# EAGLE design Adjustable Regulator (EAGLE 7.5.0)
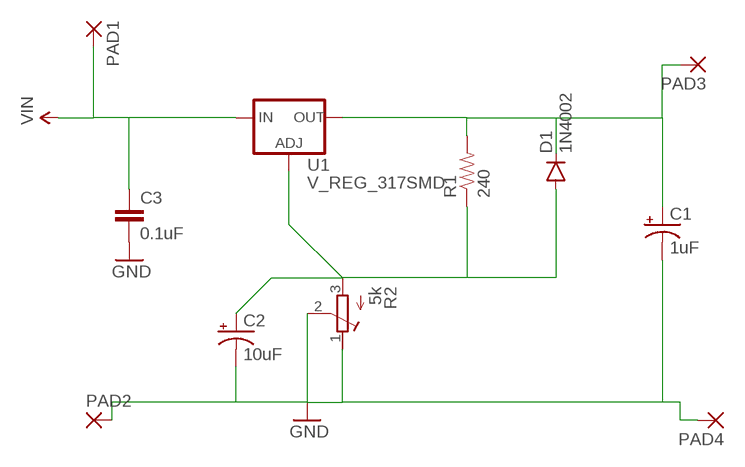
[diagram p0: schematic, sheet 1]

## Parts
C1  1uF  CAP_POLC  [PANASONIC_C]
C2  10uF  CAP_POLC  [PANASONIC_C]
C3  0.1uF  0.1UF-25V(+80/-20%)(0603)  [0603-CAP]
D1  1N4002  DIODESMB  [SMB-DIODE]
PAD1  SMD2  [SMD1,27-2,54]
PAD2  SMD2  [SMD1,27-2,54]
PAD3  SMD2  [SMD1,27-2,54]
PAD4  SMD2  [SMD1,27-2,54]
R1  240  RESISTOR0805-RES  [0805]
R2  5k  R-TRIMMT93YB  [RTRIMT93YB]
U1  V_REG_317SMD  [SOT223]

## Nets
GND: C1.- C2.- C3.2 PAD2.1(P) PAD4.1(P) R2.1(E) R2.2(S)
N$1: C2.+ D1.A R1.1 R2.3(A) U1.1(ADJ)
N$3: C1.+ D1.C PAD3.1(P) R1.2 U1.2(OUT)
VIN: C3.1 PAD1.1(P) U1.3(IN)

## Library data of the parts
C1 C2 = SparkFun-Capacitors:CAP_POL: Capacitor Polarized
C3 = SparkFun-Capacitors:0.1UF-25V(+80/-20%)(0603): CAP-00810; PROD_ID: CAP-00810
D1 = SparkFun-DiscreteSemi:DIODE: Diode; PROD_ID: DIO-09646
PAD1-PAD4 = wirepad:SMD2: SMD PAD
R1 = SparkFun-Passives:RESISTOR: Resistor
R2 = resistor:R-TRIMM: Trimm resistor
U1 = SparkFun-PowerIC:V_REG_317: Voltage Regulator Standard LM317 adjustable voltage regulator. AOI (Adjust Output Input). Google 'LM317 Calculator' for easy to use app to get the two resistor values needed. 240/720 for 5V output. 240/390 for 3.3V output. Spark Fun Electronics SKU : COM-00527

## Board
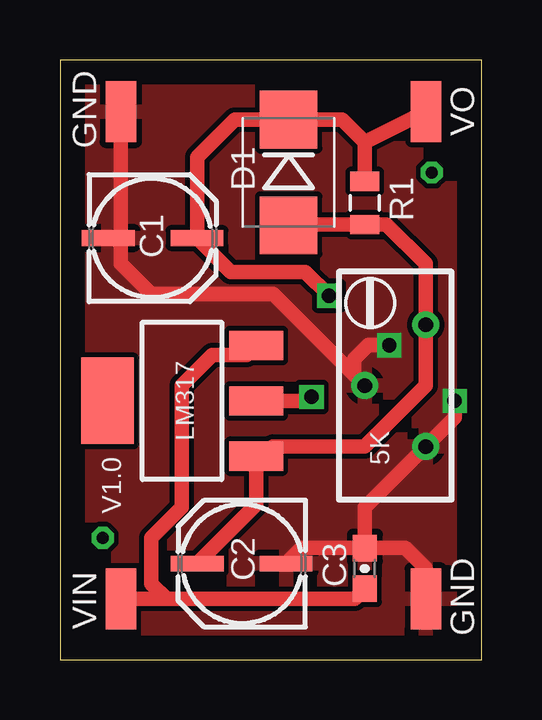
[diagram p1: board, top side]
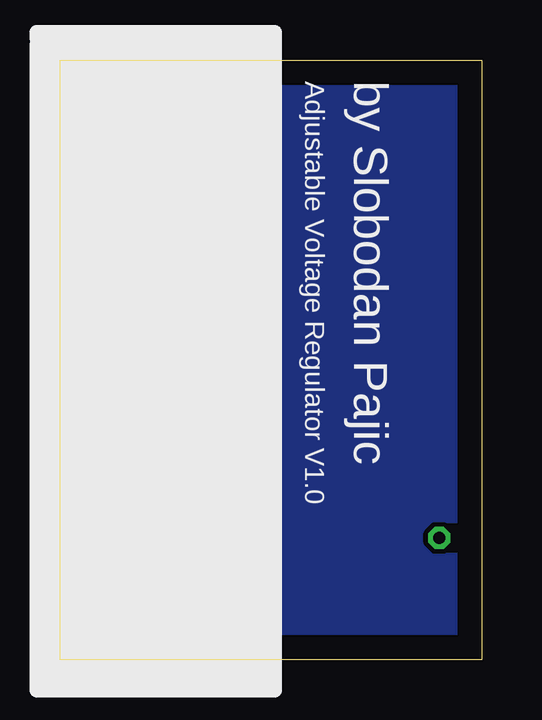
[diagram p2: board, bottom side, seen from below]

Size 17.58 x 25.01 mm. Coordinates in mm from the lower left corner, seen from the top.
Outline: 0,0 17.58,0 17.58,25.01 0,25.01 0,0
Copper layers (1*16): Top 0.035mm / dielectric 1.5mm / Bottom 0.035mm
Design rules "default": minimum track width 10mil, minimum drill 24mil, track to track 8mil, track to pad 8mil, pad to pad 8mil, via to via 8mil, smd to smd 8mil, copper to edge 40mil, drill to drill 8mil, minimum pad ring 10mil, minimum via ring 8mil, stop-mask expansion 4mil, vias tented up to drill 0mil, thermal gap 10mil

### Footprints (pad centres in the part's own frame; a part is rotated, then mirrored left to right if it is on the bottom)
PANASONIC_C = smd 2.2 x 0.65: + 1.9,-0.2; - -1.8,-0.2
0603-CAP = smd 1.1 x 1: 1 -0.85,0; 2 0.85,0
SMB-DIODE = smd 2.4 x 2.4: A 2.2,0; C -2.2,0
SMD1,27-2,54 = smd 1.27 x 2.54: 1 0,0
0805 = smd 0.8 x 1.2: 1 -0.9,0; 2 0.9,0
RTRIMT93YB = drill 0.61: 1 1.27,-2.54; 2 -1.27,0; 3 1.27,2.54
SOT223 = smd 1.219 x 2.235: 1 -2.311,-3.099; 2 0,-3.099; 3 2.311,-3.099 | smd 3.6 x 2.2: 4 0,3.099

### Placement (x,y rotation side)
C1  3.81,17.78 0 top
C2  7.62,3.81 180 top
C3  12.7,3.81 90 top
D1  9.53,20.32 270 top
PAD1  2.54,2.54 0 top
PAD2  15.24,2.54 0 top
PAD3  15.24,22.86 0 top
PAD4  2.54,22.86 0 top
R1  12.7,19.05 90 top
R2  13.97,11.43 0 top
U1  5.08,10.79 90 top

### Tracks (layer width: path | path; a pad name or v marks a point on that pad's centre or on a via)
GND  (via drill 0.6)
  Top 0.61: C3.2 14.39,4.66 15.24,3.81 PAD2.1 | C2.- 10.07,4.66 C3.2 | C3.2 12.7,6.35 R2.1 16.44,10.09 v16.44,10.79 | PAD4.1 2.54,17.78 | 2.54,17.78 2.34,17.58 C1.- | 2.54,17.78 2.54,16.51 3.81,15.24 8.89,15.24 12.27,11.87 | 12.27,11.87 R2.2 | v13.72,13.12 12.83,13.12 12.27,12.55 12.27,11.87
  Bottom 0.61: v16.44,10.79 14.12,13.12 v13.72,13.12
  pour Top: -0.76,25.91 -0.76,-1.52 19.3,-1.52 19.3,-1.27 19.56,-1.27 19.56,25.91
  pour Bottom: -1.27,25.91 -1.52,25.91 -1.52,-1.27 19.81,-1.27 19.81,-0.76 19.81,25.91
N$1
  Top 0.61: C2.+ 8.18,6.47 U1.1 8.89,8.89 12.7,8.89 15.24,11.43 R2.3 15.24,16.51 13.6,18.15 R1.1 9.55,18.15 D1.A
N$2  (via drill 0.5)
  other vias: 15.49,20.32
N$3  (via drill 0.6)
  Top 0.61: PAD3.1 12.7,21.59 | 12.7,21.59 R1.2 | 12.7,21.59 11.77,22.52 D1.C 7.28,22.52 5.71,20.95 C1.+ 7.12,16.17 10.22,16.17 v11.21,15.18 | v10.48,10.96 10.31,10.79 U1.2
  Bottom 0.61: v11.21,15.18 11.21,11.7 v10.48,10.96
N$4  (via drill 0.5)
  other vias: 1.78,5.08
VIN
  Top 0.61: C3.1 12.28,2.54 4.45,2.54 | U1.3 7.77,12.7 6.35,12.7 5.08,11.43 5.08,6.35 3.81,5.08 3.81,3.17 4.45,2.54 | 4.45,2.54 PAD1.1

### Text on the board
tNames: VO | GND | D1 | R1 | C1 | LM317 | 5K | V1.0 | C2 | C3 | VIN | GND
bNames: by Slobodan Pajic | Adjustable Voltage Regulator V1.0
